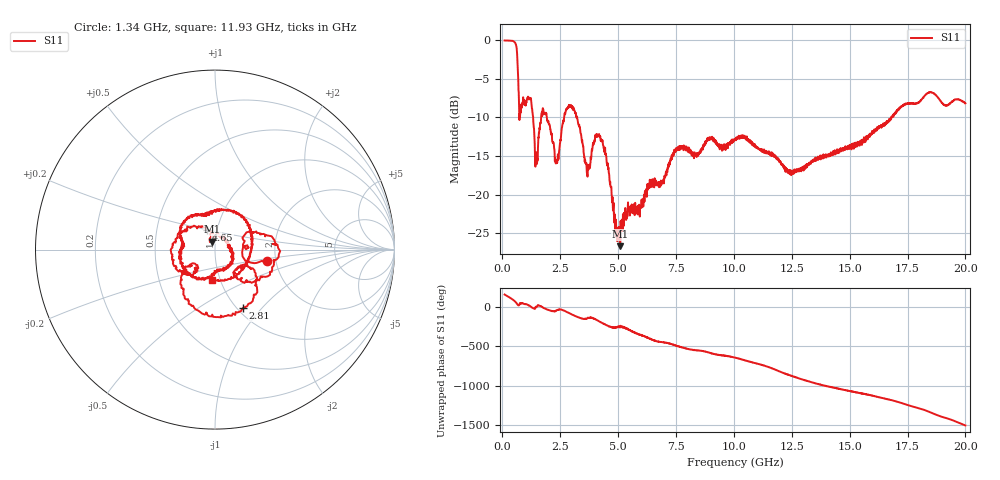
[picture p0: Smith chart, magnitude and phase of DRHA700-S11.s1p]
!Keysight Technologies,P9374A,MY57211922,A.15.40.13
!Date: Sunday, July 05, 2026 11:46:54
!Correction: S11(C  1-Port  )
!S1P File: Measurement: S11:
# Hz S  dB  R 50
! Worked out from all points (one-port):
!   1991 points, 100 MHz to 20 GHz, reference 50 ohm
!   lowest |S11| = -26.7 dB at 5.09 GHz (marker M1), VSWR 1.10, Z = 48.4 + j4.27 ohm
!   |S11| at or under -10 dB: 1.332 GHz to 1.677 GHz (345 MHz wide, 22.9 % of centre); 1.922 GHz to 2.673 GHz (750.6 MHz wide, 32.7 % of centre); 3.234 GHz to 16.8 GHz (13.56 GHz wide, 135 % of centre)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
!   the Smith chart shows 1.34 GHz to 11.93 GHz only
!   S11 on the Smith chart (normalised r, x): 1.34 GHz: 1.79, -0.25; 2.81 GHz: 1.07, -0.79; 4.65 GHz: 0.89, +0.19; 11.93 GHz: 0.92, -0.32
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1e8  -0.04 162.9
4.4e8  -0.08 101.0
6.3e8  -1.38 46.0
7.4e8  -10.34 34.0
1.34e9  -10.60 -12.6
1.48e9  -15.27 0.7
1.83e9  -9.40 -14.2
2.35e9  -15.93 -39.4
2.59e9  -11.01 -33.5
2.81e9  -8.87 -64.2
3.32e9  -10.94 -131.2
3.65e9  -17.11 -146.3
4.15e9  -12.45 -173.3
4.65e9  -18.58 113.7
5.08e9  -24.76 101.8
5.09e9  -26.67 108.4
7.57e9  -13.98 -137.3
1.005e10  -12.90 77.3
1.095e10  -13.80 4.8
1.193e10  -15.40 -94.9
1.254e10  -17.00 -160.5
1.375e10  -15.43 90.9
1.503e10  -13.95 7.5
1.672e10  -10.49 -100.3
1.752e10  -8.26 -170.4
1.857e10  -6.80 86.9
1.942e10  -7.99 -0.5
2e10  -8.17 -70.4
